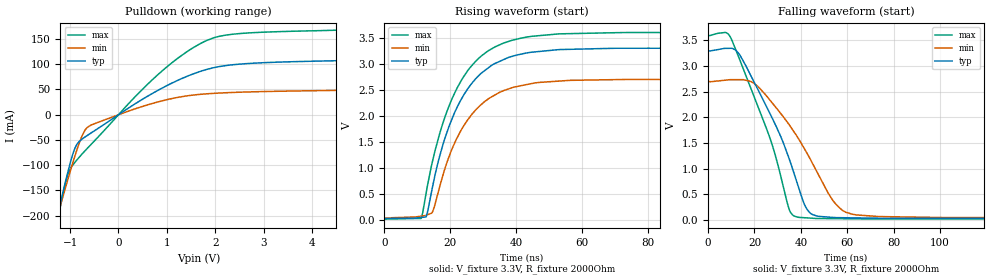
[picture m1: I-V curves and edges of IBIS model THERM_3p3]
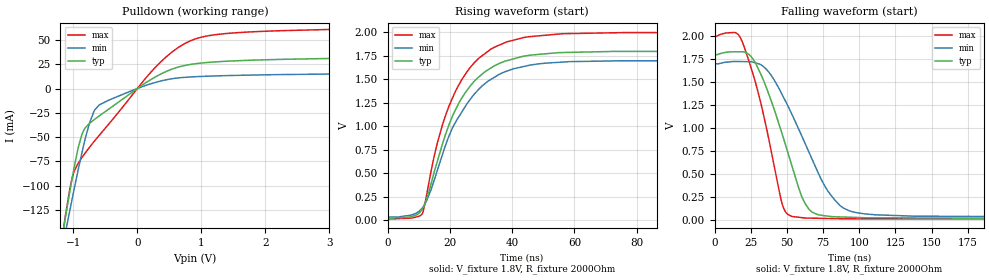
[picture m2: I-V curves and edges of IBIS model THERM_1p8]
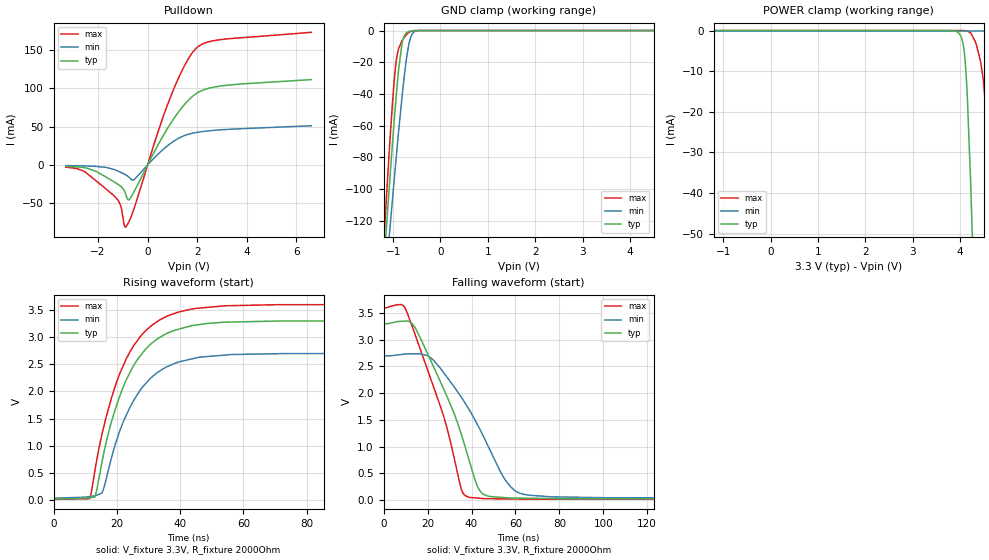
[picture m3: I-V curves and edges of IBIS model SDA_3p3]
|Texas Instruments Incorporated
| Marketing part#   Digital Voltage Range   Package-type   #pins
|  TMP9R001   1.8V - 3.3V   QFN   10
[IBIS Ver]   4.1
[File name]   tmp9r001.ibs
[File Rev]   1.0
[Date]   08/08/2025
[Source]
| Texas Instruments Incorporated.
| 12500 TI Blvd
| Dallas, TX -75243
[Notes]   Revision History:
| Rev 1.0: 04/06/2015
| - Initial version of the model
| - Model generated from simulations in TISPICE
| - C_comp although listed in numerical order of value are
|   obtained from varying PVT conditions. For PVT conditions for
|   each specific value refer the buffer description under
|   respective [Model]. IBIS model user is responsible for using
|   appropriate C_comp to simulate for Signal Integrity.
| - Warnings regarding combined Non-monotonicity of various models have been
|   reviewd and considered minor and can be ignored.
| - Model names with a trailing _1p8 contain the model for
|   1.8V operation. Model names with a trailing _3p3 contain the model
|   for 3.3V operation.
[Disclaimer]
| This model is designed as an aid for customers of Texas Instruments.
| TI and its licensors and suppliers make no warranties, either expressed
| or implied, with respect to this  model, including the warranties of
| merchantability or fitness for a particular purpose. The model is
| provided solely on an "as is" basis. The entire risk as to its quality
| and performance is with the customer.
[Copyright]
 (C) Copyright 2015 Texas Instruments Incorporated.All rights reserved.
|   Device
[Component]   TMP9R001
[Manufacturer]   TI
[Package]   |WQFN 10 pin
| variable   typ   min   max
R_pkg  6.72725E-02   6.26300E-02   8.04000E-02
L_pkg  1.72557E+00nH 1.61576E+00nH 2.00802E+00nH
C_pkg  3.04549E-01pF 2.91740E-01pF 3.15100E-01pF
[Pin]  signal_name   model_name   R_pin   L_pin   C_pin
1   V+   POWER   0.06311   1.62856nH   0.31029pF
2   D+   NC   0.06786   1.74072nH   0.29174pF
3   D-   NC   0.06786   1.74072nH   0.29174pF
4   THERMB   THERM   0.06295   1.62719nH   0.31430pF
5   A0   A   0.06268   1.63079nH   0.31241pF
6   GND   GND   0.06309   1.63746nH   0.31013pF
7   ALERTB   ALERT   0.06295   1.62719nH   0.31430pF
8   SDA   SDA   0.06295   1.62719nH   0.31430pF
9   SCL   SCL   0.08040   2.00802nH   0.30390pF
10   A1   A   0.06949   1.78291nH   0.29195pF
|   Model Selectors
[Model Selector]  SDA
SDA_3p3  SDA buffer at 3.3V operation.
SDA_1p8  SDA buffer at 1.8V operation.
[Model Selector]  SCL
SCL_3p3  SCL buffer at 3.3V operation.
SCL_1p8  SCL buffer at 1.8V operation.
[Model Selector]  A
A_3p3  Ax input buffer at 3.3V operation.
A_1p8  Ax input buffer at 1.8V operation.
[Model Selector]  THERM
THERM_3p3  THERM buffer at 3.3V operation.
THERM_1p8  THERM buffer at 1.8V operation.
[Model Selector]  ALERT
ALERT_3p3  ALERT buffer at 3.3V operation.
ALERT_1p8  ALERT buffer at 1.8V operation.
| Models and submodels in the file (10): THERM_3p3 (Open_drain), THERM_1p8 (Open_drain), SDA_3p3 (I/O_open_drain), SDA_1p8 (I/O_open_drain), SCL_3p3 (Input), SCL_1p8 (Input), ALERT_3p3 (Open_drain), ALERT_1p8 (Open_drain), A_3p3 (Input), A_1p8 (Input)
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|   Model
[Model]   THERM_3p3
Model_type   Open_drain
Polarity   Non-Inverting
Vmeas = 1.65
Vref = 3.3
Cref = 1pF
Rref = 2000
|   typ   min   max
C_comp   1.531pF   1.410pF   1.617pF
[Voltage Range]   3.3   2.7   3.6
[Temperature Range]   25   125   -40
[Pullup Reference]   3.3   2.7   3.6
[Pulldown Reference]   0   0   0
[Power Clamp Reference]   3.3   2.7   3.6
[GND Clamp Reference]   0   0   0
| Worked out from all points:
|   slope of the pulldown table from 0 to 0.495 V, typ, clamps not added: 16.2 ohm
|   falling waveform, V_fixture 3.3V, R_fixture 2000Ohm: 20-80 % time 18.4ns typ, 21.5ns min, 16.3ns max; typ from 3.3 V to 0.025 V
|   rising waveform, V_fixture 3.3V, R_fixture 2000Ohm: 20-80 % time 12.1ns typ, 12.1ns min, 12.2ns max; typ from 0.025 V to 3.3 V
[Pulldown]
|   Voltage   I(typ)   I(min)   I(max)
-3.3V     -1.116A    -955.4mA   -1.287A
-1.369V   -246mA     -238.5mA   -263.3mA
-1.261V   -199.9mA   -200.5mA   -209.5mA
-1.122V   -143mA     -153.3mA   -145.8mA
-1.033V   -108.4mA   -123.7mA   -114.7mA
-864.6mV  -59.24mA   -70.96mA   -90.14mA
-755.7mV  -48.37mA   -42.34mA   -78.08mA
-646.8mV  -41.18mA   -25.33mA   -66.84mA
848.1mV   50.03mA    26.17mA    82.24mA
1.818V    89.56mA    41.4mA     146.9mA
2.788V    102.1mA    45.41mA    162.6mA
6.6V      111.2mA    51.14mA    172.8mA
[Ramp]
R_load = 2000
|   typ   min   max
dV/dt_r   1.96491/1.20924e-08   1.59755/1.20903e-08   2.15001/1.22054e-08
dV/dt_f   1.9649/1.83658e-08   1.59748/2.14911e-08   2.15001/1.62649e-08
[Falling Waveform]
V_fixture = 3.3V
V_fixture_min = 2.7V
V_fixture_max = 3.6V
R_fixture = 2000Ohm
C_fixture = 0F
|   Time   V(typ)   V(min)   V(max)
0s        3.3V       2.7V       3.6V
9.83ns    3.348V     2.736V     3.547V
21.21ns   2.567V     2.613V     2.245V
27.83ns   1.969V     2.272V     1.438V
34.94ns   1.196V     1.859V     208.1mV
38.35ns   728.8mV    1.63V      57.03mV
44.31ns   123.5mV    1.164V     34.49mV
54.78ns   45.2mV     324.7mV    24.8mV
64.16ns   38.74mV    96.37mV    20.79mV
300ns     25.17mV    37.54mV    16.66mV
[Rising Waveform]
V_fixture = 3.3V
V_fixture_min = 2.7V
V_fixture_max = 3.6V
R_fixture = 2000Ohm
C_fixture = 0F
|   Time   V(typ)   V(min)   V(max)
0s        25.14mV    37.41mV    16.65mV
11.21ns   47.6mV     72.8mV     28.45mV
12.66ns   56.71mV    88.94mV    492.4mV
14.68ns   640.8mV    155.4mV    1.131V
17.94ns   1.47V      883.7mV    1.883V
24.23ns   2.409V     1.815V     2.761V
32.52ns   2.965V     2.36V      3.282V
41.88ns   3.188V     2.582V     3.495V
73.56ns   3.297V     2.697V     3.598V
300ns     3.3V       2.7V       3.6V
|   Model
[Model]   THERM_1p8
Model_type   Open_drain
Polarity   Non-Inverting
Vmeas = 0.9
Vref = 1.8
Cref = 1pF
Rref = 2000
|   typ   min   max
C_comp   1.531pF   1.410pF   1.617pF
[Voltage Range]   1.8   1.7   2
[Temperature Range]   25   125   -40
[Pullup Reference]   1.8   1.7   2
[Pulldown Reference]   0   0   0
[Power Clamp Reference]   1.8   1.7   2
[GND Clamp Reference]   0   0   0
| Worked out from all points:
|   slope of the pulldown table from 0 to 0.27 V, typ, clamps not added: 23.5 ohm
|   falling waveform, V_fixture 1.8V, R_fixture 2000Ohm: 20-80 % time 21.9ns typ, 29.8ns min, 17.2ns max; typ from 1.8 V to 0.019 V
|   rising waveform, V_fixture 1.8V, R_fixture 2000Ohm: 20-80 % time 13ns typ, 14.1ns min, 12.6ns max; typ from 0.019 V to 1.8 V
[Pulldown]
|   Voltage   I(typ)   I(min)   I(max)
-1.8V     -422.9mA   -392.3mA   -467.2mA
-1.195V   -162.2mA   -173.7mA   -163.8mA
-1.125V   -133.9mA   -149.6mA   -131.9mA
-1.049V   -104.4mA   -124.2mA   -102mA
-995.4mV  -84.54mA   -106.6mA   -87.17mA
-865.8mV  -47.54mA   -66.49mA   -71.33mA
-747mV    -35.93mA   -35.57mA   -60.56mA
-595.8mV  -28.29mA   -16.95mA   -48.32mA
273.6mV   11.64mA    6.12mA     21.26mA
743.4mV   23.8mA     11.54mA    46.41mA
1.445V    28.28mA    13.4mA     56.98mA
3.6V      31.71mA    15.37mA    61.83mA
[Ramp]
R_load = 2000
|   typ   min   max
dV/dt_r   1.06867/1.29941e-08   1.00015/1.40574e-08   1.19298/1.26504e-08
dV/dt_f   1.06863/2.19161e-08   0.999951/2.96221e-08   1.19297/1.72245e-08
[Falling Waveform]
V_fixture = 1.8V
V_fixture_min = 1.7V
V_fixture_max = 2V
R_fixture = 2000Ohm
C_fixture = 0F
|   Time   V(typ)   V(min)   V(max)
0s        1.8V       1.7V       2V
13.71ns   1.829V     1.724V     2.039V
18.77ns   1.83V      1.723V     1.948V
32.9ns    1.551V     1.678V     1.205V
46.21ns   957.7mV    1.377V     200.7mV
52.48ns   637.2mV    1.18V      46.11mV
65.67ns   109.5mV    721.2mV    22.05mV
78.8ns    42.4mV     304.5mV    17.62mV
94.37ns   30.85mV    95.2mV     14.86mV
300ns     18.94mV    33.41mV    11.72mV
[Rising Waveform]
V_fixture = 1.8V
V_fixture_min = 1.7V
V_fixture_max = 2V
R_fixture = 2000Ohm
C_fixture = 0F
|   Time   V(typ)   V(min)   V(max)
0s        18.88mV    33.08mV    11.71mV
11.22ns   122.3mV    131.1mV    72.09mV
15.08ns   525.6mV    437.7mV    697.5mV
17.7ns    820.2mV    707mV      1.024V
20.89ns   1.112V     987.4mV    1.306V
25.6ns    1.388V     1.245V     1.586V
32.28ns   1.602V     1.482V     1.8V
43.64ns   1.746V     1.637V     1.945V
75.38ns   1.798V     1.698V     1.998V
300ns     1.8V       1.7V       2V
|   Model
[Model]   SDA_3p3
Model_type   I/O_open_drain
Polarity   Non-Inverting
Enable   Active-Low
Vinl = 0.99
Vinh = 2.31
Vmeas = 1.65
Vref = 3.3
Cref = 1pF
Rref = 2000
|   typ   min   max
C_comp   1.538pF   1.417pF   1.633pF
[Voltage Range]   3.3   2.7   3.6
[Temperature Range]   25   125   -40
[Pullup Reference]   3.3   2.7   3.6
[Pulldown Reference]   0   0   0
[Power Clamp Reference]   3.3   2.7   3.6
[GND Clamp Reference]   0   0   0
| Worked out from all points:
|   slope of the pulldown table from 0 to 0.495 V, typ, clamps not added: 16.2 ohm
|   GND clamp passes 1 mA (typ) near -0.70 V on its own axis
|   falling waveform, V_fixture 3.3V, R_fixture 2000Ohm: 20-80 % time 18.4ns typ, 21.5ns min, 16.3ns max; typ from 3.3 V to 0.025 V
|   rising waveform, V_fixture 3.3V, R_fixture 2000Ohm: 20-80 % time 12ns typ, 12.1ns min, 12.2ns max; typ from 0.025 V to 3.3 V
[Pulldown]
|   Voltage   I(typ)   I(min)   I(max)
-3.3V     -1.776mA   -825uA     -2.828mA
-2.577V   -3.361mA   -1.225mA   -8.028mA
-1.31V    -22.85mA   -6.418mA   -41.48mA
-1.092V   -27.65mA   -9.509mA   -52.46mA
-884.4mV  -38.02mA   -12.85mA   -80.99mA
-686.4mV  -42.87mA   -18.02mA   -69.16mA
-518.1mV  -33.07mA   -18.25mA   -53.88mA
986.7mV   57.03mA    29.48mA    93.69mA
1.511V    79.69mA    38.6mA     130.8mA
1.957V    92.95mA    42.29mA    152mA
2.927V    102.8mA    45.74mA    163.2mA
6.6V      111.2mA    51.14mA    172.8mA
[GND Clamp]
|   Voltage   I(typ)   I(min)   I(max)
-3.3V     -1.114A    -954.5mA   -1.284A
-1.191V   -145.8mA   -168.7mA   -130.6mA
-1.122V   -116.1mA   -144.2mA   -95.81mA
-1.073V   -95.26mA   -126.9mA   -72.01mA
-983.4mV  -59.42mA   -96.41mA   -33.98mA
-933.9mV  -41.05mA   -79.94mA   -19.09mA
-884.4mV  -24.79mA   -63.95mA   -11.42mA
-815.1mV  -8.701mA   -42.82mA   -6.687mA
-676.5mV  -703.3uA   -10.1mA    -1.463mA
-597.3mV  -154.5uA   -2.214mA   -337.7uA
-448.8mV  -5.051uA   -45.02uA   -7.672uA
6.6V      0A         0A         0A
[POWER Clamp]
|   Voltage   I(typ)   I(min)   I(max)
-3.3V     0A         1.065nA    0A
3.877V    -102.2uA   0A         -51.72nA
4.066V    -3.442mA   0A         -12.64uA
4.115V    -8.701mA   0A         -48.25uA
4.155V    -16.69mA   0A         -128.4uA
4.224V    -37.59mA   0A         -584.6uA
4.323V    -75.02mA   0A         -2.756mA
4.501V    -150.1mA   0A         -13.32mA
4.561V    -176.1mA   0A         -26.27mA
4.6V      -193.6mA   0A         -40.37mA
4.65V     -215.5mA   0A         -61.51mA
6.6V      -1.114A    0A         -1.118A
[Ramp]
R_load = 2000
|   typ   min   max
dV/dt_r   1.96491/1.19924e-08   1.59755/1.19865e-08   2.15001/1.21644e-08
dV/dt_f   1.9649/1.83702e-08   1.59747/2.14921e-08   2.15001/1.62707e-08
[Falling Waveform]
V_fixture = 3.3V
V_fixture_min = 2.7V
V_fixture_max = 3.6V
R_fixture = 2000Ohm
C_fixture = 0F
|   Time   V(typ)   V(min)   V(max)
0s        3.3V       2.7V       3.6V
10.23ns   3.347V     2.734V     3.55V
22.63ns   2.501V     2.617V     2.127V
29.03ns   1.92V      2.288V     1.318V
35.38ns   1.229V     1.924V     203.8mV
38.47ns   806.4mV    1.722V     60.2mV
44.86ns   127.9mV    1.241V     33.11mV
55.26ns   47.73mV    381.6mV    25.03mV
65.86ns   37.87mV    95.09mV    20.16mV
300ns     25.17mV    37.54mV    16.66mV
[Rising Waveform]
V_fixture = 3.3V
V_fixture_min = 2.7V
V_fixture_max = 3.6V
R_fixture = 2000Ohm
C_fixture = 0F
|   Time   V(typ)   V(min)   V(max)
0s        25.14mV    37.41mV    16.65mV
11.43ns   48.32mV    67.23mV    27.92mV
13.06ns   57.74mV    82.14mV    539mV
15.51ns   759.8mV    156.4mV    1.266V
18.24ns   1.432V     763.4mV    1.866V
24.74ns   2.419V     1.773V     2.787V
32.6ns    2.959V     2.339V     3.279V
42.65ns   3.195V     2.585V     3.505V
73.86ns   3.297V     2.698V     3.597V
300ns     3.3V       2.7V       3.6V
